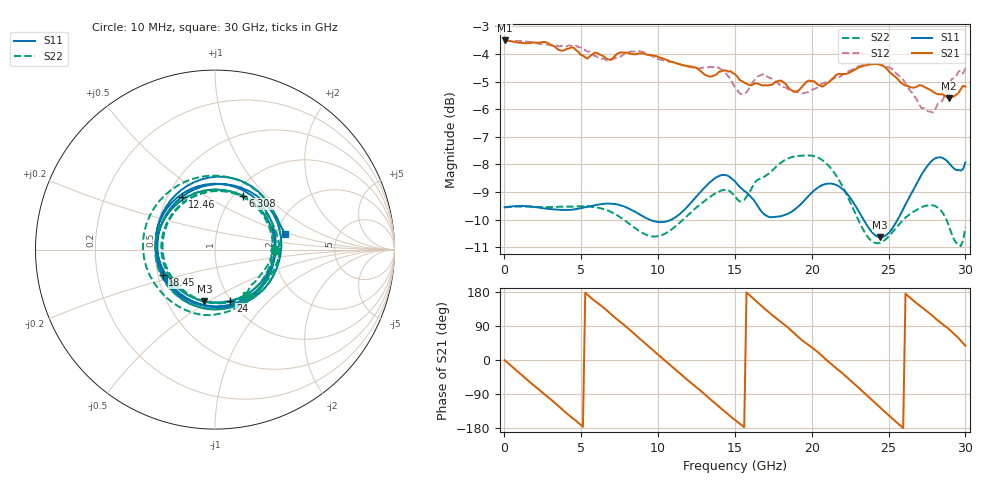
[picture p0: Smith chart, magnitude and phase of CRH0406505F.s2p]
#HZ S MA R 50
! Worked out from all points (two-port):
!   201 points, 10 MHz to 30 GHz, reference 50 ohm
!   highest |S21| = -3.51 dB at 10 MHz (marker M1); lowest = -5.6 dB at 28.95 GHz (marker M2)
!   |S21| within 3 dB of the highest: start of sweep to end of sweep
!   lowest |S11| = -10.6 dB at 24.45 GHz (marker M3), VSWR 1.83, Z = 37.9 - j23.9 ohm
!   |S11| at or under -10 dB: 9.43 GHz to 10.87 GHz (1.44 GHz wide, 14.2 % of centre); 23.36 GHz to 25.59 GHz (2.229 GHz wide, 9.11 % of centre)
!   |S22| runs from -11.0 to -7.7 dB; largest |S21 - S12| = 0.056
!   S11 on the Smith chart (normalised r, x): 10 MHz: 2.00, -0.01; 6.308 GHz: 1.11, +0.75; 12.46 GHz: 0.59, +0.40; 18.45 GHz: 0.53, -0.17; 24 GHz: 0.99, -0.62; 30 GHz: 2.22, +0.46
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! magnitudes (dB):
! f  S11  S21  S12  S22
! 10 MHz  -9.6  -3.5  -3.5  -9.6
! 5.108 GHz  -9.6  -4.1  -3.8  -9.5
! 6.308 GHz  -9.4  -4.0  -4.2  -9.6
! 8.707 GHz  -9.8  -4.0  -3.9  -10.4
! 10.06 GHz  -10.1  -4.1  -4.2  -10.6
! 12.46 GHz  -9.2  -4.5  -4.5  -9.6
! 13.81 GHz  -8.5  -4.7  -4.5  -9.0
! 15.01 GHz  -8.6  -4.7  -5.2  -9.2
! 15.6 GHz  -9.0  -5.0  -5.4  -9.3
! 17.1 GHz  -9.9  -5.1  -4.8  -8.4
! 18.45 GHz  -9.8  -5.2  -5.3  -7.8
! 20.1 GHz  -9.0  -5.0  -5.3  -7.7
! 20.7 GHz  -8.7  -5.2  -5.1  -7.9
! 21.9 GHz  -8.9  -4.7  -4.8  -8.7
! 24 GHz  -10.5  -4.4  -4.4  -10.8
! 24.45 GHz  -10.6  -4.4  -4.4  -10.8
! 25.05 GHz  -10.5  -4.6  -4.5  -10.6
! 27.6 GHz  -8.0  -5.3  -6.1  -9.5
! 28.35 GHz  -7.7  -5.5  -5.8  -9.6
! 28.95 GHz  -8.0  -5.6  -5.1  -10.3
! 29.7 GHz  -8.2  -5.3  -4.6  -11.0
! 30 GHz  -7.9  -5.2  -4.5  -10.3
